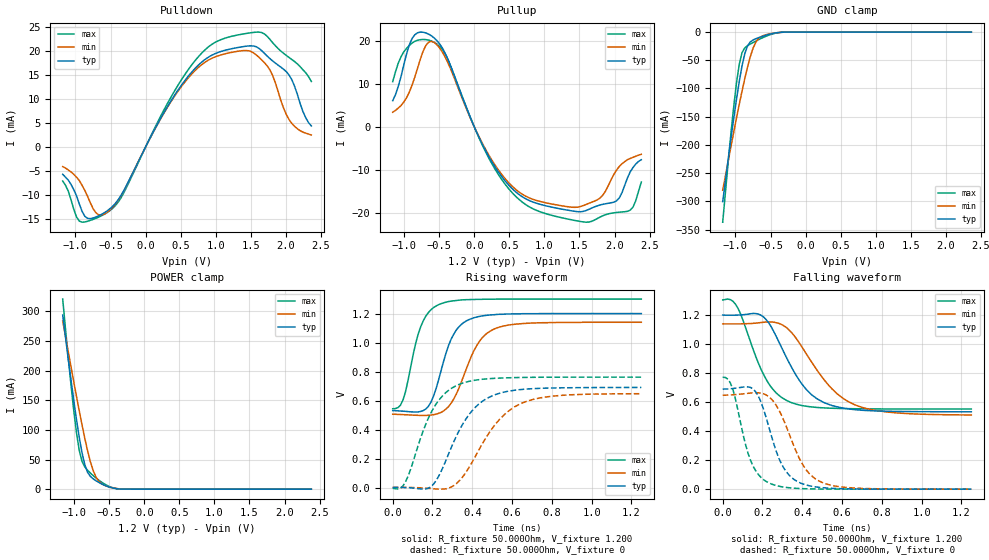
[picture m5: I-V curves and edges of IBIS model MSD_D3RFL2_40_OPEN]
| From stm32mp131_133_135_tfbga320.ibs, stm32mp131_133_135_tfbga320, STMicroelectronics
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[Model] MSD_D3RFL2_40_OPEN
Model_type   I/O
C_comp 2.581pF   2.493pF   2.708pF
Vinh = 820.000mV
Vinl = 380.000mV
Vmeas = 600.000mV
Vref = 600.000mV
[Model Spec]
Vinh   820.000mV   790.000mV   870.000mV
Vinl   380.000mV   350.000mV   430.000mV
Vmeas   600.000mV   570.000mV   650.000mV
Vref   600.000mV   570.000mV   650.000mV
[Receiver Thresholds]
Vth   =  0.600V
Vth_min  =  0.5880V
Vth_max  =  0.6120V
Vinh_ac  =  0.220V
Vinh_dc  =  0.130V
Vinl_ac  = -0.220V
Vinl_dc  = -0.130V
Tslew_ac =  5.000ns |Not specified, so set to high value
[Temperature Range]   25.000   125.000   -40.000
[Voltage Range]   1.200V   1.140V   1.300V
[GND Clamp Reference]   0.00V   0.00V   0.00V
[Pulldown Reference]   0.00V   0.00V   0.00V
[POWER Clamp Reference]   1.200V   1.140V   1.300V
[Pullup Reference]   1.200V   1.140V   1.300V
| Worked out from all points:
|   slope of the pulldown table from 0 to 0.18 V, typ, clamps not added: 35.6 ohm
|   slope of the pullup table from 0 to 0.18 V, typ, clamps not added: 29.6 ohm
|   GND clamp passes 1 mA (typ) near -0.40 V on its own axis
|   POWER clamp passes 1 mA (typ) near -0.41 V on its own axis
|   rising waveform, R_fixture 50.000Ohm, V_fixture 1.200: 20-80 % time 97ps typ, 124ps min, 83.4ps max; typ from 0.531 V to 1.2 V
|   rising waveform, R_fixture 50.000Ohm, V_fixture 0: 20-80 % time 162ps typ, 194ps min, 140ps max; typ from 0.001 V to 0.69 V
|   falling waveform, R_fixture 50.000Ohm, V_fixture 1.200: 20-80 % time 171ps typ, 212ps min, 139ps max; typ from 1.2 V to 0.533 V
|   falling waveform, R_fixture 50.000Ohm, V_fixture 0: 20-80 % time 106ps typ, 129ps min, 89.9ps max; typ from 0.69 V to 0 V
[GND Clamp]
-1.182V   -300.5mA   -280.4mA   -337mA
-1.064V   -188.1mA   -202.5mA   -178.5mA
-984.9mV  -118.6mA   -152.2mA   -89.49mA
-945.5mV  -87.16mA   -127.9mA   -56.6mA
-906.1mV  -59.71mA   -104.4mA   -36.4mA
-866.7mV  -38.14mA   -82.14mA   -27.92mA
-827.3mV  -24.29mA   -61.54mA   -24.05mA
-748.5mV  -14mA      -28.45mA   -18.47mA
-709.1mV  -11.76mA   -17.8mA    -15.89mA
-630.3mV  -8.132mA   -7.75mA    -11.05mA
-472.7mV  -2.557mA   -2.242mA   -3.323mA
2.364V    29.58nA    484.6nA    2.864nA
[Power Clamp]
-1.164V   293.6mA    283.6mA    320.6mA
-1.085V   219.6mA    231.9mA    221.3mA
-1.006V   149.3mA    180.9mA    132.2mA
-966.7mV  116.7mA    156mA      94.33mA
-927.3mV  86.87mA    131.6mA    64.9mA
-887.9mV  61.07mA    108mA      46.71mA
-809.1mV  28.38mA    64.84mA    31.83mA
-730.3mV  17.49mA    31.58mA    22.97mA
-651.5mV  11.58mA    13.7mA     15.38mA
-533.3mV  4.956mA    4.897mA    6.46mA
-336.4mV  215.7uA    403.7uA    242.8uA
2.382V    -24.83nA   -515.5nA   -2.721nA
[Pulldown]
-1.182V   -5.7mA     -4.1mA     -7.1mA
-945.5mV  -11.89mA   -7mA       -15.47mA
-866.7mV  -14.47mA   -9.06mA    -15.65mA
-709.1mV  -14.63mA   -13.73mA   -14.9mA
-551.5mV  -13.38mA   -13.65mA   -13.72mA
-354.6mV  -10.22mA   -10.29mA   -10.71mA
590.9mV   14.46mA    14.13mA    15.79mA
945.5mV   19.18mA    18.53mA    21.44mA
1.339V    20.84mA    20.05mA    23.47mA
1.733V    19.01mA    16.97mA    23.14mA
2.009V    15.71mA    6.73mA     19.1mA
2.364V    4.4mA      2.5mA      13.7mA
[Pullup]
-1.164V   6.1mA      3.409mA    10.51mA
-887.9mV  20.51mA    9.705mA    19.46mA
-730.3mV  21.96mA    17.56mA    20.29mA
-612.1mV  21.14mA    19.85mA    19.94mA
-375.8mV  15.68mA    14.87mA    15.58mA
215.2mV   -7.105mA   -6.743mA   -7.481mA
727.3mV   -16.61mA   -16.01mA   -17.94mA
1.515V    -19.67mA   -18.45mA   -21.93mA
1.791V    -18.11mA   -16.51mA   -20.92mA
1.988V    -17.46mA   -11.08mA   -19.92mA
2.264V    -9.4mA     -7.043mA   -18.57mA
2.382V    -7.6mA     -6.348mA   -12.78mA
[Ramp]
R_load=50.000Ohm
dV/dt_r   407.310mV/130.000ps  383.549mV/159.500ps  452.790mV/112.000ps
dV/dt_f   407.310mV/139.500ps  383.518mV/172.000ps  452.790mV/115.000ps
[Rising waveform]
R_fixture=50.000Ohm
V_fixture=1.200
V_fixture_min=1.140
V_fixture_max=1.300
0s        531mV      506mV      543.3mV
52ps      526.6mV    502.8mV    604.7mV
128ps     521.7mV    498mV      1.058V
166ps     541.6mV    497.3mV    1.181V
230ps     739.6mV    511.4mV    1.261V
281ps     980.2mV    558.4mV    1.283V
332ps     1.107V     682.9mV    1.292V
422ps     1.176V     978.2mV    1.298V
511ps     1.192V     1.094V     1.299V
1.25ns    1.2V       1.14V      1.3V
[Rising waveform]
R_fixture=50.000Ohm
V_fixture=0
0s        805uV      842.6uV    -5.173mV
64ps      104.4uV    762.2uV    38.47mV
192ps     5.311mV    -7.096mV   514.4mV
243ps     110.3mV    -11.26mV   620.7mV
320ps     354.1mV    26.5mV     702.9mV
447ps     591.1mV    293mV      746.3mV
537ps     650.2mV    469.6mV    754.9mV
639ps     675.3mV    575.4mV    759mV
843ps     687.6mV    635.3mV    761.2mV
1.25ns    690.4mV    647.2mV    761.5mV
[Falling waveform]
R_fixture=50.000Ohm
V_fixture=1.200
V_fixture_min=1.140
V_fixture_max=1.300
0s        1.2V       1.139V     1.304V
77ps      1.2V       1.139V     1.246V
205ps     1.187V     1.15V      791.5mV
269ps     1.053V     1.147V     663.1mV
345ps     842.9mV    1.081V     596.7mV
473ps     624mV      822.3mV    563.3mV
575ps     567.5mV    657.6mV    556.6mV
652ps     549.8mV    589.2mV    554.5mV
830ps     537mV      531.1mV    552.6mV
1.25ns    533.1mV    511.3mV    552.2mV
[Falling waveform]
R_fixture=50.000Ohm
V_fixture=0
0s        689.8mV    647.5mV    771.3mV
52ps      693.6mV    650.4mV    683.4mV
115ps     705.1mV    658.7mV    306.1mV
154ps     689.3mV    663.9mV    155.8mV
230ps     438.4mV    638.8mV    44.72mV
281ps     217.3mV    549.1mV    20.83mV
332ps     99.61mV    388.6mV    9.929mV
409ps     33.3mV     154.6mV    3.272mV
498ps     10.82mV    47.46mV    935.2uV
1.25ns    7.551uV    39.02uV    2.44uV
